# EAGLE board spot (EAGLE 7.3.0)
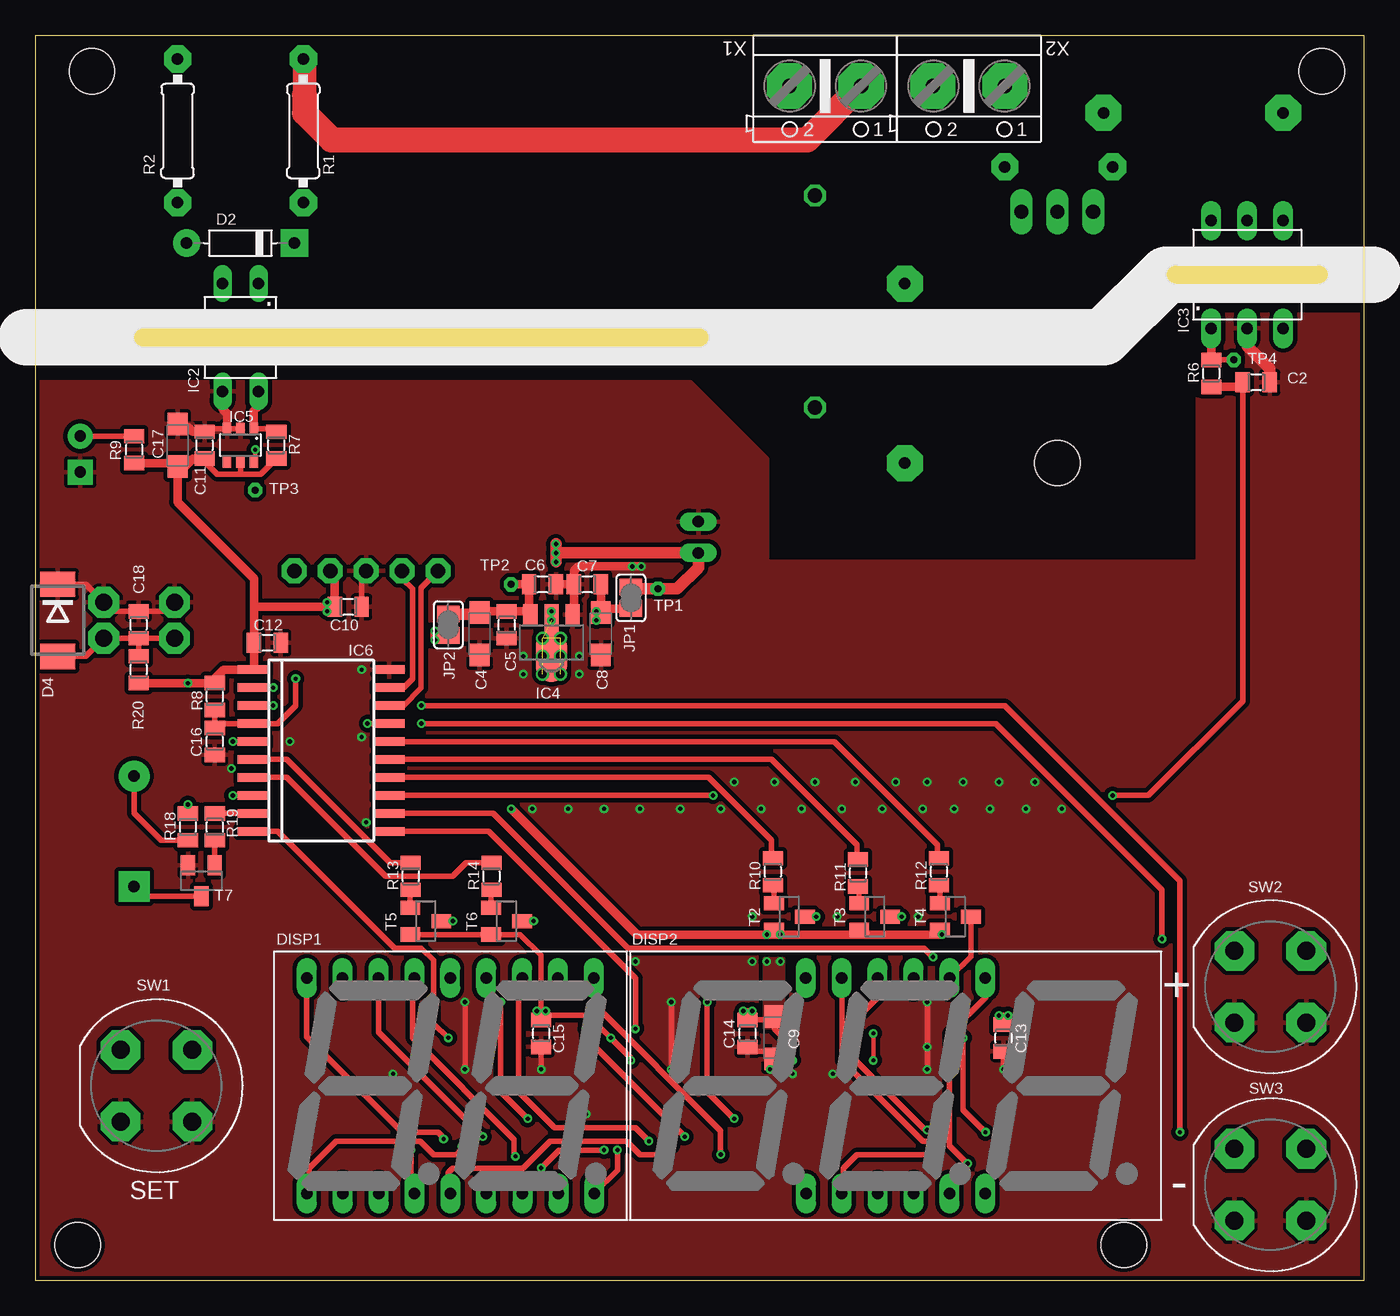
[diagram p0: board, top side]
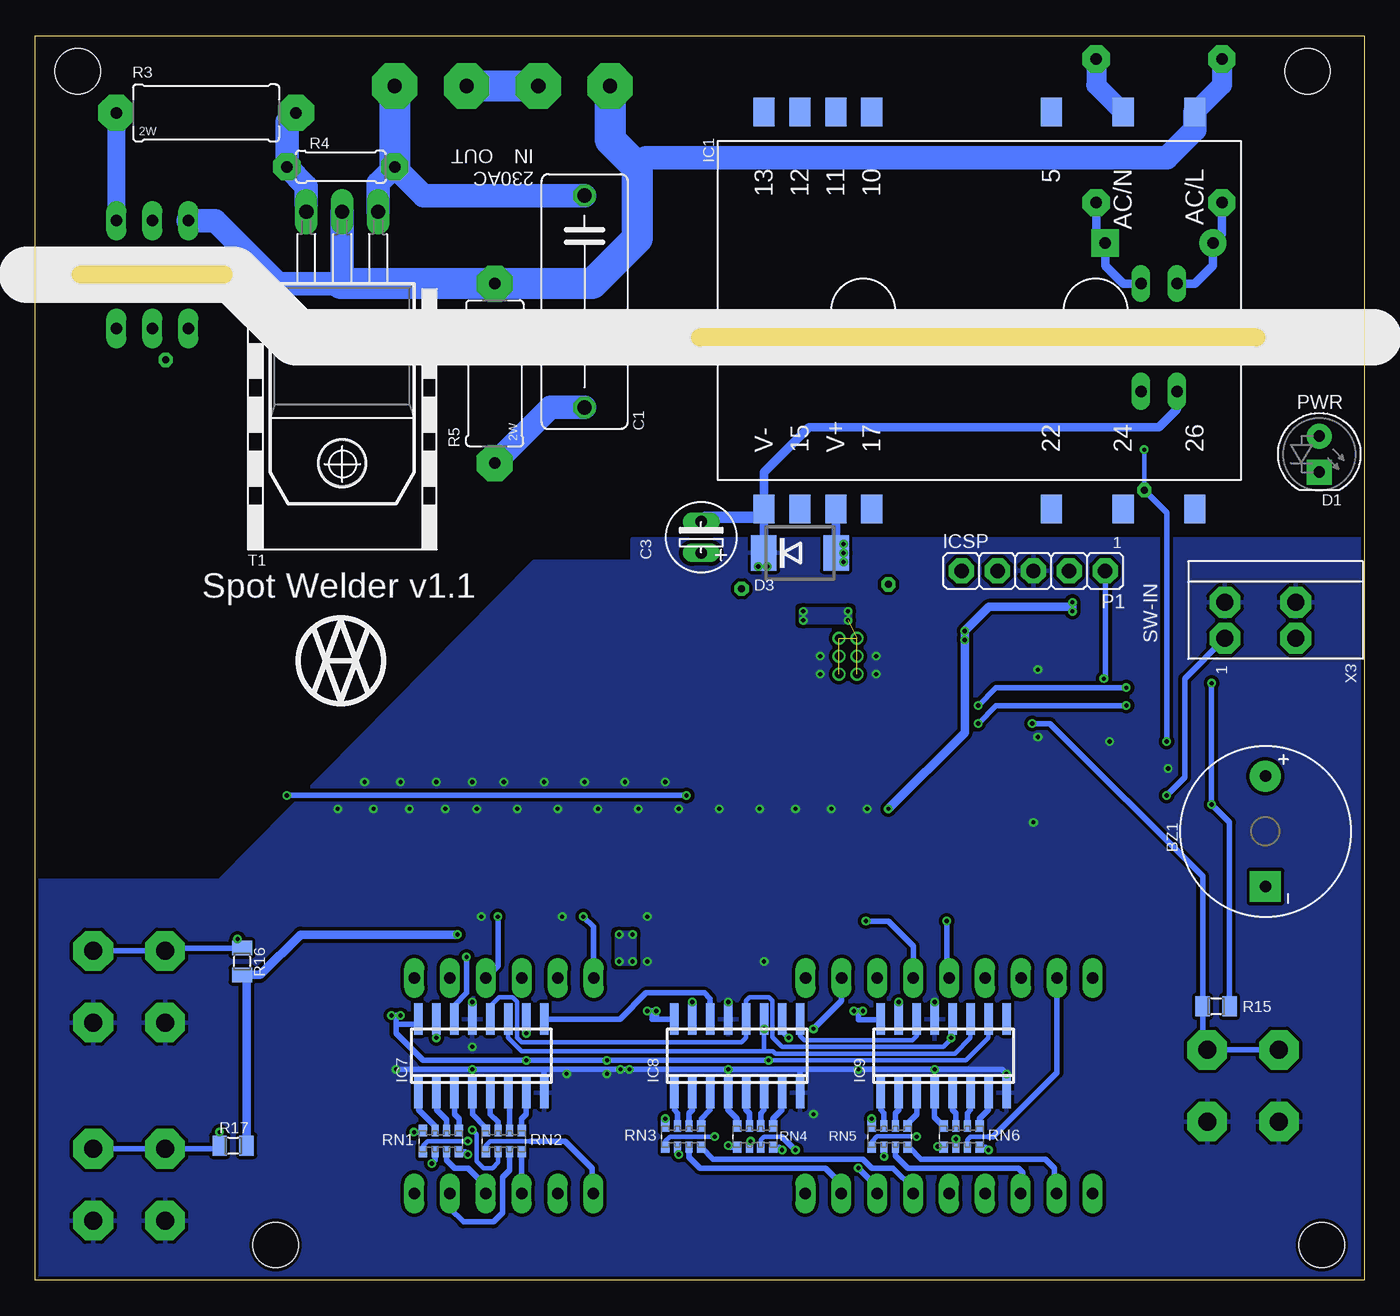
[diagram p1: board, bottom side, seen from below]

Size 94 x 88 mm. Coordinates in mm from the lower left corner, seen from the top.
Outline: 0,0 94,0 94,88 0,88 0,0
Copper layers (1*16): Top 0.035mm / dielectric 1.5mm / Bottom 0.035mm
Design rules "ITEADstudio_DRC": minimum track width 6mil, minimum drill 12mil, track to track 6mil, track to pad 6mil, pad to pad 6mil, via to via 6mil, smd to smd 0mil, copper to edge 10mil, drill to drill 10mil, minimum pad ring 10mil, minimum via ring 6mil, stop-mask expansion 2mil, vias tented up to drill 100mil, thermal gap 10mil
Holes 3.2 mm at 4,85.5 77,2.5 3,2.5 91,85.5 72.3,57.8
Milling: 2 lines

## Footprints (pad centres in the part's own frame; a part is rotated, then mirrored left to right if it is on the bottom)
BZEG1205 = drill 0.813 pad 2.184: + -3.9,0 | drill 0.813 pad 2.184 square: - 3.9,0
C150-064X183 = drill 1.016 octagon: 1 -7.493,0; 2 7.493,0
0805 = smd 1.016 x 1.422: 1 -0.953,0; 2 0.953,0
C-EL_2 = drill 0.813 pad 1.27 long: C+ 0,0; C- 2.223,0
SMC_A = smd 1.6 x 1.4: + -1.5,0; - 1.5,0
LED_5 = drill 0.813 pad 1.778: A -1.27,0 | drill 0.813 pad 1.778 square: K 1.27,0
DO35 = drill 0.813 pad 1.93: A -3.81,0 | drill 0.813 pad 1.93 square: K 3.81,0
DO214AA = smd 1.8 x 2.5: A 2.55,0; K -2.55,0
OPD-2 = drill 0.813 pad 1.4 long: 1 -10.16,-7.62; 2 -7.62,-7.62; 3 -5.08,-7.62; 4 -2.54,-7.62; 5 0,-7.62; 6 2.53,-7.62; 7 5.09,-7.62; 8 7.63,-7.62; 9 10.17,-7.62; 10 10.15,7.62; 11 7.61,7.62; 12 5.07,7.62; 13 2.53,7.62; 14 -0.01,7.62; 15 -2.55,7.62; 16 -5.09,7.62; 17 -7.63,7.62; 18 -10.17,7.62
OPD-3 = drill 0.813 pad 1.4 long: 1 -6.35,-7.62; 2 -3.81,-7.62; 3 -1.27,-7.62; 4 1.27,-7.62; 5 3.81,-7.62; 6 6.34,-7.62; 7 6.34,7.62; 8 3.8,7.62; 9 1.26,7.62; 10 -1.28,7.62; 11 -3.82,7.62; 12 -6.36,7.62
IRM_03_SMD = smd 1.5 x 2.03: 5 -5.08,-14.035; 10 7.62,-14.035; 11 10.16,-14.035; 12 12.7,-14.035; 13 15.24,-14.035; 15 12.7,14.035; 17 7.62,14.035; 22 -5.08,14.035; 24 -10.16,14.035; 26 -15.24,14.035; AC/L -15.24,-14.035; AC/N -10.16,-14.035; V+ 10.16,14.035; V- 15.24,14.035
DIL4 = drill 0.813 pad 1.27 long: 1 -1.27,-3.81; 2 1.27,-3.81; 3 1.27,3.81; 4 -1.27,3.81
DIL6 = drill 0.813 pad 1.4 long: 1 -2.54,-3.81; 2 0,-3.81; 3 2.54,-3.81; 4 2.54,3.81; 5 0,3.81; 6 -2.54,3.81
SOT89 = smd 1 x 1.5: 1 -1.499,-1.981; 3 1.499,-1.981 | smd 1 x 2: 2 0,-1.727 | smd 2.2 x 3.7: 2@1 0,0.94
SOT23-6 = smd 0.6 x 0.9: 1 -0.95,-1.15; 2 0,-1.15; 3 0.95,-1.15; 4 0.95,1.15; 5 0,1.15; 6 -0.95,1.15
SO-20 = smd 0.6 x 2.2: 1 -5.715,-4.8; 2 -4.445,-4.8; 3 -3.175,-4.8; 4 -1.905,-4.8; 5 -0.635,-4.8; 6 0.635,-4.8; 7 1.905,-4.8; 8 3.175,-4.8; 9 4.445,-4.8; 10 5.715,-4.8; 11 5.715,4.8; 12 4.445,4.8; 13 3.175,4.8; 14 1.905,4.8; 15 0.635,4.8; 16 -0.635,4.8; 17 -1.905,4.8; 18 -3.175,4.8; 19 -4.445,4.8; 20 -5.715,4.8
SO-16 = smd 0.6 x 2.2: 1 -4.445,-2.917; 2 -3.175,-2.917; 3 -1.905,-2.917; 4 -0.635,-2.917; 5 0.635,-2.917; 6 1.905,-2.917; 7 3.175,-2.917; 8 4.445,-2.917; 9 4.445,2.283; 10 3.175,2.283; 11 1.905,2.283; 12 0.635,2.283; 13 -0.635,2.283; 14 -1.905,2.283; 15 -3.175,2.283; 16 -4.445,2.283
JP = smd 1.168 x 1.6: 1 -0.762,0; 2 0.762,0
S5G1 = drill 1.016 pad 1.778 octagon: 1 -5.08,0; 2 -2.54,0; 3 0,0; 4 2.54,0; 5 5.08,0
R-10 = drill 0.813 pad 1.93 octagon: 1 -5.08,0; 2 5.08,0
R-_2W = drill 0.813 pad 2.54 octagon: 1 -6.35,0; 2 6.35,0
R-7,5 = drill 0.813 pad 1.93 octagon: 1 -3.81,0; 2 3.81,0
EXB38V = smd 0.6 x 0.8: 1 -1.275,-0.75; 4 1.275,-0.75; 5 1.275,0.75; 8 -1.275,0.75 | smd 0.5 x 0.8: 2 -0.4,-0.75; 3 0.4,-0.75; 6 0.4,0.75; 7 -0.4,0.75
P-DT6 = drill 1.27 pad 2.8 octagon: 1 -2.54,-2.54; 1A -2.54,2.54; 2 2.54,-2.54; 2A 2.54,2.54
TO-220 = drill 1.016 pad 1.6 long: 1 -2.54,0; 2 0,0; 3 2.54,0
SOT23 = smd 1 x 1.4: 1 -0.95,-1.1; 2 0.95,-1.1; 3 0,1.1
PAD_0,8 = drill 0.5 pad 0.813 octagon: 1 0,0
ARK500/2 = drill 1 pad 3.2 octagon: 1 -2.54,0; 2 2.54,0
DG240W = drill 1.2 pad 2.184 octagon: 1 -1.27,-2.54; 1_1 -1.27,2.46; 2 1.27,-2.54; 2_2 1.27,2.46

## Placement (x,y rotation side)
BZ1  BZEG-1205  [BZEG1205]  6.99,31.75 270 bottom
C1  100n/630  [C150-064X183]  55.15,69.22 270 bottom
C2  1n  [0805]  86.36,63.5 0 top
C3  47u/10  [C-EL_2]  46.9,51.44 90 bottom
C4  47u/6.3  [SMC_A]  31.43,45.72 270 top
C5  10u/10  [0805]  33.34,46.35 270 top
C6  100n  [0805]  35.88,49.21 0 top
C7  100n  [0805]  39.05,49.21 180 top
C8  10u/10  [SMC_A]  40.01,45.72 270 top
C9  10u/10  [SMC_A]  52.29,17.14 270 top
C10  100n  [0805]  22.13,47.62 0 top
C11  100n  [0805]  11.97,59.05 90 top
C12  100n  [0805]  16.41,45.09 0 top
C13  100n  [0805]  68.48,17.14 270 top
C14  100n  [0805]  50.39,17.46 270 top
C15  100n  [0805]  35.78,17.46 270 top
C16  100n  [0805]  12.7,38.1 270 top
C17  10u/10  [SMC_A]  10.06,59.05 90 top
C18  10n  [0805]  7.3,46.35 90 top
D1  [LED_5]  3.17,58.42 270 bottom
D2  1N4148  [DO35]  14.51,73.34 0 top
D3  P6SMBJ  [DO214AA]  39.91,51.44 0 bottom
D4  P6SMBJ  [DO214AA]  1.59,46.67 270 top
DISP1  OPD-D5630UPG  [OPD-2]  29.36,13.76 0 top
DISP2  OPD-T5620LE  [OPD-3]  60.87,13.76 0 top
IC1  [IRM_03_SMD]  27.21,68.58 180 bottom
IC2  PC817  [DIL4]  14.51,66.67 180 top
IC3  MOC3020  [DIL6]  85.72,71.12 0 top
IC4  MCP1702  [SOT89]  36.51,45.09 180 top
IC5  7417  [SOT23-6]  14.51,59.05 180 top
IC6  PIC16F18344SOIC  [SO-20]  20.23,37.47 270 top
IC7  74595SO  [SO-16]  62.45,16.19 0 bottom
IC8  74595SO  [SO-16]  44.35,16.19 0 bottom
IC9  74595SO  [SO-16]  29.75,16.19 0 bottom
JP1  JP  [JP]  42.13,48.26 90 top
JP2  JP  [JP]  29.21,46.35 270 top
KK1  D0A-L  [D02A-L]  72.3,63.18 90 bottom
P1  ICSP  [S5G1]  23.4,50.16 180 bottom
R1  100k  [R-10]  18.95,81.28 90 top
R2  100k  [R-10]  10.06,81.28 90 top
R3  1k  [R-_2W]  81.92,82.55 0 bottom
R4  330  [R-7,5]  72.39,78.74 180 bottom
R5  100  [R-_2W]  61.5,64.14 90 bottom
R6  1k  [0805]  83.19,64.14 90 top
R7  10k  [0805]  17.05,59.05 90 top
R8  10k  [0805]  12.7,41.27 90 top
R9  1k  [0805]  6.99,58.74 270 top
R10  2k  [0805]  52.17,28.89 90 top
R11  2k  [0805]  58.2,28.79 90 top
R12  2k  [0805]  63.92,28.89 90 top
R13  2k  [0805]  26.55,28.57 90 top
R14  2k  [0805]  32.27,28.57 90 top
R15  10k  [0805]  10.48,19.37 0 bottom
R16  10k  [0805]  79.38,22.54 270 bottom
R17  10k  [0805]  80.01,9.53 0 bottom
R18  220  [0805]  10.79,32.07 90 top
R19  10k  [0805]  12.7,32.07 270 top
R20  10k  [0805]  7.3,43.18 270 top
RN1  1k  [EXB38V]  65.31,9.84 0 bottom
RN2  1k  [EXB38V]  60.87,9.84 0 bottom
RN3  10k  [EXB38V]  48.16,10.16 0 bottom
RN4  10k  [EXB38V]  43.09,10.16 0 bottom
RN5  10k  [EXB38V]  33.56,10.16 0 bottom
RN6  10k  [EXB38V]  28.48,10.16 0 bottom
SW1  P-DT6  [P-DT6]  8.56,13.76 90 top
SW2  P-DT6  [P-DT6]  87.36,20.76 90 top
SW3  P-DT6  [P-DT6]  87.36,6.76 90 top
T1  BTA140  [TO-220]  72.3,75.56 180 bottom
T2  BC857  [SOT23]  53.34,25.72 270 top
T3  BC857  [SOT23]  59.37,25.72 270 top
T4  BC857  [SOT23]  65.09,25.72 270 top
T5  BC857  [SOT23]  27.62,25.4 270 top
T6  BC857  [SOT23]  33.34,25.4 270 top
T7  BC847  [SOT23]  11.75,28.26 180 top
TP1  PAD_10,8  [PAD_0,8]  44.04,48.9 0 top
TP2  PAD_10,8  [PAD_0,8]  33.66,49.21 0 top
TP3  PAD_10,8  [PAD_0,8]  15.56,55.88 0 top
TP4  PAD_10,8  [PAD_0,8]  84.77,65.09 0 top
U$1  [LOGO_AV3]  72.39,43.81 0 top
X1  AC IN  [ARK500/2]  55.88,84.45 180 top
X2  AC OUT  [ARK500/2]  66.04,84.45 180 top
X3  HANDLE  [DG240W]  7.3,46.67 270 bottom

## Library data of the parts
BZ1 C2 C3 C5-C7 C10-C16 C18 D1 IC2 R1-R20 T1 TP1-TP4 = #PaJa_31
C1 C4 C8 C9 C17 = rcl
D2 IC3 = #PaJa_30
D3 D4 IC4-IC9 JP1 JP2 P1 T2-T7 U$1 = !mcom2a
DISP1 DISP2 = #PaJa_displeje
IC1 = meanwell_irm_v7
KK1 = heatsink
RN1-RN6 = resistor-dil; OC_FARNELL: unknown; OC_NEWARK: unknown
SW1-SW3 = #PaJa_prepinace
X1-X3 = #PaJa_konektory

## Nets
!MCLR: C16.1 IC6.4 P1.1 R8.1
+3,3V: C9.+ C10.1 C11.1 C12.1 C13.1 C14.1 C15.1 C17.+ IC5.5 IC6.1 IC7.10 IC7.16 IC8.10 IC8.16 IC9.10 IC9.16 JP2.2 P1.2 R7.1 R8.2 R9.2 R15.2 R16.2 R17.2 R18.2 R20.2 T2.2 T3.2 T4.2 T5.2 T6.2
+5V: C3.C+ D3.A IC1.V+ JP1.2 TP1.1
BEEP: IC6.9 R19.1
CAD1_1: IC6.14 R10.2
CAD1_2: IC6.15 R11.2
CAD1_3: IC6.16 R12.2
CAD2_1: IC6.6 R13.2
CAD2_2: IC6.7 R14.2
D1_CA1: DISP2.12 T2.3
D1_CA2: DISP2.9 T3.3
D1_CA3: DISP2.8 T4.3
D2_CA1: DISP1.14 T5.3
D2_CA2: DISP1.13 T6.3
DS: IC6.12 IC7.14
GND: C2.2 C3.C- C4.- C5.2 C6.2 C7.2 C8.- C9.- C10.2 C11.2 C12.2 C13.2 C14.2 C15.2 C16.2 C17.- C18.2 D1.K D3.K D4.K IC1.V- IC2.3 IC3.2 IC4.1 IC5.2 IC5.3 IC6.20 IC7.8 IC7.13 IC8.8 IC8.13 IC9.8 IC9.13 P1.3 SW1.1 SW1.1A SW2.1 SW2.1A SW3.1 SW3.1A T7.2 X3.1 X3.1_1
INPUT: C18.1 D4.A IC6.8 R20.1 X3.2 X3.2_2
N$1: D2.K IC2.1 R1.1
N$2: D2.A IC2.2 R2.1
N$4: IC7.15 RN1.8
N$5: IC8.9 IC9.14
N$6: IC1.AC/L IC3.6 R2.2 R5.2 T1.2 X1.2
N$7: IC3.4 R3.1
N$8: R3.2 R4.2 T1.3
N$9: C1.1 R4.1 T1.1 X2.1
N$10: IC3.1 R6.2 TP4.1
N$11: C7.1 C8.+ IC4.2 JP1.1
N$12: C1.2 R5.1
N$13: C4.+ C5.1 C6.1 IC4.3 JP2.1 TP2.1
N$14: IC7.9 IC8.14
N$15: IC7.4 RN2.8
N$16: IC7.1 RN1.7
N$17: IC7.2 RN1.6
N$18: IC7.5 RN2.7
N$19: IC7.6 RN2.6
N$20: IC7.7 RN2.5
N$21: IC7.3 RN1.5
N$22: DISP2.11 RN1.1
N$23: DISP2.7 RN1.2
N$24: DISP2.4 RN1.3
N$25: DISP2.2 RN1.4
N$26: DISP2.1 RN2.1
N$27: DISP2.10 RN2.2
N$28: DISP2.5 RN2.3
N$29: DISP2.3 RN2.4
N$30: IC8.1 RN3.7
N$31: IC8.2 RN3.6
N$32: IC8.5 RN4.7
N$33: IC8.6 RN4.6
N$34: IC8.7 RN4.5
N$35: IC8.3 RN3.5
N$36: DISP1.16 RN5.1
N$37: DISP1.15 RN5.2
N$38: DISP1.3 RN5.3
N$39: DISP1.2 RN5.4
N$40: DISP1.1 RN6.1
N$41: DISP1.18 RN6.2
N$42: DISP1.17 RN6.3
N$43: DISP1.4 RN6.4
N$44: IC9.1 RN5.7
N$45: IC9.2 RN5.6
N$46: IC9.5 RN6.7
N$47: IC9.6 RN6.6
N$48: IC9.7 RN6.5
N$49: IC9.3 RN5.5
N$50: DISP1.11 RN3.1
N$51: DISP1.10 RN3.2
N$52: DISP1.8 RN3.3
N$53: DISP1.6 RN3.4
N$54: DISP1.5 RN4.1
N$55: DISP1.12 RN4.2
N$56: DISP1.7 RN4.3
N$57: DISP1.9 RN4.4
N$58: IC8.15 RN3.8
N$59: IC8.4 RN4.8
N$60: IC9.15 RN5.8
N$61: IC9.4 RN6.8
N$62: D1.A R9.1
N$63: R10.1 T2.1
N$64: R11.1 T3.1
N$65: R12.1 T4.1
N$66: R13.1 T5.1
N$67: R14.1 T6.1
N$68: BZ1.+ R18.1
N$69: BZ1.- T7.3
N$70: R19.2 T7.1
N$72: IC1.AC/N R1.2 X1.1 X2.2
N$74: IC2.4 IC5.1 R7.2
PGC: IC6.18 P1.5
PGD: IC6.19 P1.4
SCTP: IC6.10 IC7.12 IC8.12 IC9.12
SHCP: IC6.11 IC7.11 IC8.11 IC9.11
START: C2.1 IC6.13 R6.1
SW+: IC6.3 R16.1 SW2.2 SW2.2A
SW-: IC6.2 R17.1 SW3.2 SW3.2A
SW_P: IC6.17 R15.1 SW1.2 SW1.2A
ZERO: IC5.6 IC6.5 TP3.1

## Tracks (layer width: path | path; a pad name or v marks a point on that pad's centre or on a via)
!MCLR  (via drill 0.3)
  Top 0.406: R8.1 C16.1 13.02,39.37 IC6.4 17.14,39.37 18.41,40.64 v18.41,42.55
  Bottom 0.406: P1.1 18.32,42.64 v18.41,42.55
+3,3V  (via drill 0.3)
  Top 0.305: v59.28,17.46 v59.28,15.56
  Top 0.406: 36.1,18.73 v36.1,19.05 v35.47,19.05 35.76,19.05 35.77,19.06 35.77,22.97 34.29,24.45 T6.2 T5.2 | 36.1,18.73 35.78,18.73 C15.1 | v42.13,15.56 42.13,15.72 v40.7,17.14 39.12,18.73 36.1,18.73 | v50.7,19.05 v50.07,19.05 50.07,18.41 C14.1 52.06,18.41 C9.+ 52.29,17.78 53.56,16.51 v53.56,15.56 | v68.8,18.73 v68.17,18.73 68.48,18.73 C13.1 | JP2.2 28.57,45.59 v28.26,45.28 | R18.2 v10.79,33.66 | 17.05,58.01 R7.1 15.94,56.99 14.61,56.99 | IC5.5 14.51,57.09 14.61,56.99 | C11.1 11.97,57.88 12.86,56.99 14.61,56.99
  Top 0.61: v52.7,24.45 52.56,24.77 T2.2 | 52.07,18.87 C9.+ | C10.1 21.18,49.85 P1.2 | v28.26,45.92 v28.26,45.28 | C10.1 20.95,47.62 v20.64,47.94 v20.64,47.31 | 15.46,47.62 C10.1 | 15.46,47.62 C12.1 15.46,43.22 IC6.1 13.34,43.18 12.7,42.55 R8.2 v10.79,42.23 R20.2 | v33.66,33.34 42.55,24.45 v52.7,24.45 | T2.2 52.07,24.77 v51.75,24.45 | 15.46,47.62 15.46,49.62 10.06,55.02 C17.+ | T2.2 52.38,24.77 v52.7,24.45 | T4.2 63.99,24.45 v64.14,24.45 58.27,24.45 T3.2 58.27,24.59 58.42,24.45 v52.7,24.45 | C11.1 11.11,58.1 10.48,57.47 10.15,57.47 C17.+ | R9.2 9.84,57.78 C17.+
  Bottom 0.305: IC9.10 26.57,17.14 28.16,15.56 v42.13,15.56 | 41.18,19.21 IC8.10 41.08,18.57 41.08,17.68 | IC7.10 v59.28,17.46
  Bottom 0.406: v36.1,19.05 v35.47,19.05 35.78,19.05 C15.1 34.26,18.41 IC9.16 34.2,18.41 | 41.08,17.68 41.08,17.52 v40.7,17.14 | 50.39,19.05 v50.07,19.05 50.07,18.73 | 50.39,19.05 v50.7,19.05 | IC8.16 50.39,18.48 50.39,19.05 | C13.1 66.9,18.1 IC7.16 | C13.1 68.48,17.46 66.58,15.56 v59.28,15.56 v53.56,15.56 v42.13,15.56 | v68.17,18.73 68.48,18.73 | 68.48,18.73 v68.8,18.73 | C13.1 68.48,18.73 | v10.79,42.23 v10.79,33.66 | 10.48,33.34 v10.79,33.66 | R15.2 9.53,32.38 v10.79,33.66
  Bottom 0.61: v20.64,47.94 20.64,47.62 | 20.64,47.62 v20.64,47.31 | v28.26,45.92 28.26,45.4 | 20.64,47.62 26.55,47.62 v28.26,45.92 | v28.26,45.92 28.26,38.73 v33.66,33.34 | R17.2 79.06,21.27 R16.2 78.11,21.59 75.25,24.45 v64.14,24.45
  other vias: 51.75,22.54 52.7,22.54
  pour Bottom: 51.75,24.45 51.75,22.54 52.7,22.54 52.7,24.45
  pour Top (no thermals): 51.5,22.8 53,22.8 53,17.8 51.5,17.8
+5V  (via drill 0.3)
  Top 0.813: v36.83,51.44 v36.83,50.8 | v36.83,52.07 v36.83,51.44 | JP1.2 42.26,48.9 TP1.1 45.4,48.9 46.9,50.39 C3.C+ v36.83,51.44
  Bottom 0.61: IC1.V+ D3.A
  Bottom 0.813: 37.47,52.07 37.47,51.44 D3.A v36.83,51.44
BEEP
  Top 0.406: R19.1 IC6.9
CAD1_1
  Top 0.406: R10.2 52.07,29.95 52.07,31.11 47.62,35.56 IC6.14
CAD1_2
  Top 0.406: R11.2 58.1,29.84 58.1,30.8 52.07,36.83 IC6.15
CAD1_3
  Top 0.406: R12.2 63.82,29.95 63.82,30.8 56.52,38.1 IC6.16
CAD2_1
  Top 0.406: R13.2 25.08,29.53 17.78,36.83 IC6.6
CAD2_2
  Top 0.406: R14.2 30.48,29.53 29.53,28.57 24.77,28.57 17.78,35.56 IC6.7
D1_CA1  (via drill 0.3)
  Top 0.406: v55.24,25.72 T2.3
  Bottom 0.406: DISP2.12 54.52,25 v55.24,25.72
D1_CA2  (via drill 0.3)
  Top 0.406: v61.28,25.72 T3.3
  Bottom 0.406: v61.28,25.72 61.28,22.25 DISP2.9
D1_CA3
  Top 0.406: T4.3 66.19,22.89 DISP2.8
D2_CA1  (via drill 0.3)
  Top 0.406: v29.53,25.4 T5.3
  Bottom 0.406: v29.53,25.4 29.53,21.55 DISP1.14
D2_CA2  (via drill 0.3)
  Top 0.406: v35.24,25.4 T6.3
  Bottom 0.406: DISP1.13 31.89,23.64 33.66,25.4 v35.24,25.4
DS  (via drill 0.3)
  Top 0.406: v63.5,22.86 62.87,23.5 41.91,23.5 32.38,33.02 IC6.12
  Bottom 0.406: v63.5,22.86 63.5,20.32 64.36,19.46 IC7.14
GND  (via drill 0.3)
  Top 0.406: v44.99,19.68 v44.99,14.92 | v30.39,19.68 v30.39,14.92 | C15.2 v35.78,14.92 | v63.09,19.68 v63.09,14.92 | C13.2 v68.48,14.92 | C14.2 50.7,16.51 51.02,16.19 51.74,16.19 C9.- 52.61,15.33 v52.61,14.92 v51.98,14.92 | C10.2 23.08,49.85 P1.3 | X3.1 9.21,47.31 C18.2 5.48,47.31 X3.1_1 3.56,49.22 D4.K | IC5.2 IC5.3 12.17,60.2 C11.2
  Top 0.61: C7.2 C6.2 | C7.2 38.1,47.15 IC4.1 | v42.86,50.48 38.42,50.48 38.1,50.16 C7.2 | IC5.3 13.56,61.27 13.24,61.59 IC2.3 | C11.2 11.11,60.01 10.79,60.33 10.29,60.33 C17.-
  Top 0.813: IC3.2 85.72,66.04 87.31,64.45 C2.2
  Bottom 0.406: IC8.13 v44.99,19.68 | IC9.13 v30.39,19.68 | IC7.13 v63.09,19.68 | v68.48,14.92 v63.09,14.92 58.01,14.92 | 58.01,14.92 v51.98,14.92 v44.99,14.92 39.91,14.92 | 39.91,14.92 v35.78,14.92 v30.39,14.92 25.62,14.92 v25.3,14.61 IC9.8 | IC8.8 39.91,14.92 | IC7.8 58.01,14.92
  Bottom 0.61: IC2.3 13.24,61.59 14.51,60.33 39.27,60.33 42.45,57.15 IC1.V- 42.45,53.98 D3.K | D3.K | D3.K 42.45,50.9 v42.86,50.48
  Bottom 0.813: 42.45,53.98 46.58,53.98 C3.C-
  other vias: 42.23,50.48 56.42,14.61 53.56,14.61 38.96,11.75 63.09,16.51 23.4,32.38 23.08,38.42 18,38.1 23.08,43.18 34.51,44.13 34.51,42.86 38.48,42.86 38.48,44.13 50.7,25.72 56.74,25.72 62.45,25.72 13.88,36.2 72.61,33.34 70.71,35.24 70.07,33.34 68.17,35.24 67.53,33.34 65.63,35.24 64.99,33.34 63.09,35.24 62.77,33.34 60.87,35.24 59.91,33.34 58.01,35.24 57.05,33.34 55.15,35.24 54.2,33.34 52.29,35.24 51.34,33.34 49.44,35.24 48.48,33.34 45.62,33.34 42.77,33.34 40.23,33.34 37.69,33.34 35.15,33.34 50.7,22.54 42.45,22.54
  pour Top (isolate 0.305, rank 2): 93.98,68.26 82.23,68.26 82.23,50.8 51.75,50.8 51.75,58.1 46.35,63.5 0,63.5 0,0 93.98,0
  pour Bottom (isolate 0.254, rank 2): 0,52.39 51.75,52.39 51.75,50.8 58.74,50.8 80.96,28.26 93.98,28.26 93.98,0 0,0
INPUT  (via drill 0.3)
  Top 0.406: C18.1 R20.1 | C18.1 X3.2_2 3.56,44.12 D4.A | IC6.8 v13.97,34.29 | C18.1 X3.2
  Bottom 0.406: v13.97,34.29 12.7,35.56 12.7,42.55 X3.2
N$1
  Bottom 0.61: IC2.1 17.05,70.48 18.32,71.75 D2.K 18.95,73.98 R1.1
N$2
  Bottom 0.61: IC2.2 11.97,70.48 10.7,71.75 D2.A 10.06,73.98 R2.1
N$4  (via drill 0.3)
  Top 0.406: v65.63,17.14 65.63,12.06 v67.22,10.48
  Bottom 0.406: IC7.15 v65.63,17.14 | v67.22,10.48 66.7,10.48 RN1.8
N$5
  Bottom 0.305: IC8.9 39.91,17.3 39.59,16.99 31.97,16.99 31.66,17.3 IC9.14
N$6
  Bottom 1.422: R2.2 10.06,84.52 IC1.AC/L
  Bottom 1.676: IC1.AC/L 11.97,81.38 13.97,79.38 50.8,79.38 51.44,78.74 | 72.3,70.48 72.39,70.48 | 72.39,70.48 76.83,70.48 81.28,74.93 IC3.6 | T1.2 72.3,70.58 72.39,70.48
  Bottom 2.184: 72.39,70.48 R5.2 54.61,70.48 51.44,73.66 51.44,78.74 53.34,80.64 X1.2
N$7
  Bottom 1.27: R3.1 IC3.4
N$8
  Bottom 1.27: T1.3 74.83,76.11
  Bottom 1.676: 74.83,76.11 74.83,77.38 R4.2 76.2,81.92 R3.2
N$9
  Bottom 1.676: C1.1 66.55,76.71 R4.1 69.75,77.56 T1.1
  Bottom 2.184: X2.1 R4.1
N$10
  Top 0.406: TP4.1 R6.2
  Top 0.61: IC3.1 R6.2
N$11  (via drill 0.3, 0.6)  (6 unrouted)
  Top 0.61: C7.1 40.01,47.54 v39.69,47.31 C8.+ 40.28,47.5 JP1.1 | IC4.2 v36.51,46.67
  other vias: 36.51,47.31 39.69,46.67 35.88,45.4 37.15,45.4 35.88,44.13 37.15,44.13 35.88,42.86 37.15,42.86
  pour Bottom: 36.51,47.31 39.69,47.31 39.69,46.67 36.51,46.67
N$12
  Bottom 1.676: C1.2 57.56,61.72 R5.1
N$13
  Top 0.61: C4.+ 31.74,47.31 C5.1 34.99,47.31 IC4.3 34.92,47.15 C6.1 TP2.1
  Top 0.813: JP2.1 31.33,47.12 C4.+
N$14
  Bottom 0.406: IC7.9 52.65,18.48 50.8,20.32 46.67,20.32 46.26,19.91 IC8.14
N$15
  Bottom 0.406: RN2.8 62.14,10.8 63.09,11.75 IC7.4
N$16
  Bottom 0.406: RN1.7 65.71,10.88 66.9,12.06 IC7.1
N$17
  Bottom 0.406: IC7.2 65.63,12.06 64.91,11.35 RN1.6
N$18
  Bottom 0.406: RN2.7 61.27,11.2 61.82,11.75 IC7.5
N$19
  Bottom 0.406: RN2.6 60.47,13.19 IC7.6
N$20
  Bottom 0.406: RN2.5 59.59,11.44 59.28,11.75 IC7.7
N$21
  Bottom 0.406: IC7.3 64.36,11.75 64.04,11.43 RN1.5
N$22  (via drill 0.3)
  Top 0.406: v63.41,9.84 62.77,9.84 57.06,15.55 DISP2.11
  Bottom 0.305: RN1.1 66.58,9.52 66.26,9.84 v63.41,9.84
N$23  (via drill 0.3)
  Top 0.406: v65.94,8.26 64.67,9.53 64.67,17.46 67.22,20.01 DISP2.7
  Bottom 0.406: RN1.2 65.71,8.49 v65.94,8.26
N$24
  Bottom 0.406: RN1.3 64.91,8.49 64.36,7.94 63.41,7.94 62.16,6.69 DISP2.4
N$25  (via drill 0.3)
  Top 0.406: v63.41,8.89 58.1,8.89 57.15,7.94 57.15,6.22 DISP2.2
  Bottom 0.406: RN1.4 63.61,9.09 v63.41,8.89
N$26
  Bottom 0.305: RN2.1 62.14,9.52 61.82,9.84 58.96,9.84
  Bottom 0.406: 58.96,9.84 56.52,9.84 54.61,7.94 54.61,6.22 DISP2.1
N$27  (via drill 0.3)
  Top 0.406: v63.09,10.64 62.93,10.64 58.01,15.56 58.01,18.41 59.6,20.01 DISP2.10
  Bottom 0.305: RN2.2 61.27,8.33 61.66,7.94 62.29,7.94 62.77,8.41 62.77,10.32 v63.09,10.64
N$28
  Bottom 0.406: DISP2.5 64.69,5.1 63.72,4.13 61.59,4.13 60.96,4.76 60.96,7.3 60.47,7.8 RN2.3
N$29
  Bottom 0.406: RN2.4 59.59,6.38 DISP2.3
N$30
  Bottom 0.406: RN3.7 48.56,11.83 48.8,12.06 IC8.1
N$31
  Bottom 0.406: RN3.6 47.77,11.83 47.53,12.06 IC8.2
N$32
  Bottom 0.406: RN4.7 43.48,11.83 43.72,12.06 IC8.5
N$33
  Bottom 0.406: RN4.6 42.69,11.83 42.45,12.06 IC8.6
N$34
  Bottom 0.406: IC8.7 41.18,12.06 41.81,11.43 RN4.5
N$35
  Bottom 0.406: RN3.5 46.89,11.44 46.26,12.06 IC8.3
N$36  (via drill 0.3)
  Top 0.406: DISP1.16 24.27,17.54 v31.66,10.16
  Bottom 0.305: RN5.1 34.84,9.8 34.47,10.17 v31.66,10.17 v31.66,10.16
N$37  (via drill 0.3)
  Top 0.406: 33.96,8.88 v33.97,8.77 33.88,8.86 33.88,9.94 26.67,17.14 26.67,21.25 DISP1.15
  Bottom 0.406: v33.97,8.77 RN5.2
N$38
  Bottom 0.406: RN5.3 33.16,8.81 32.29,7.94 24.45,7.94 24.13,7.62 24.13,6.3 DISP1.3
N$39
  Bottom 0.406: RN5.4 32.17,9.41 31.34,8.57 22.54,8.57 21.91,7.94 21.91,6.31 DISP1.2
N$40  (via drill 0.3)
  Top 0.406: v30.16,9.47 30.16,9.3 29.75,8.89 28.16,8.89 27.21,9.84 21.27,9.84 19.37,7.94 19.37,6.31 DISP1.1
  Bottom 0.406: RN6.1 30.11,9.41 v30.16,9.47
N$41  (via drill 0.3)
  Top 0.406: v28.88,9.98 28.88,10.08 28.48,10.48 25.94,10.48 19.2,17.22 DISP1.18
  Bottom 0.406: RN6.2 v28.88,9.98 28.86,9.87
N$42
  Bottom 0.305: RN6.3 28.08,9.93 27.84,10.16 26.57,10.16
  Bottom 0.406: 26.57,10.16 26.26,10.16 21.73,14.68 DISP1.17
N$43  (via drill 0.3)
  Top 0.406: v26.57,9.21 26.57,6.4 DISP1.4
  Bottom 0.406: RN6.4 26.78,9.41 v26.57,9.21
N$44
  Bottom 0.406: RN5.7 33.96,11.83 34.2,12.06 IC9.1
N$45
  Bottom 0.406: RN5.6 33.16,11.83 32.92,12.06 IC9.2
N$46
  Bottom 0.406: RN6.7 28.88,11.83 29.11,12.06 IC9.5
N$47
  Bottom 0.406: RN6.6 28.08,11.83 27.84,12.06 IC9.6
N$48
  Bottom 0.406: RN6.5 27.2,11.44 26.57,12.06 IC9.7
N$49
  Bottom 0.406: RN5.5 32.28,11.12 31.66,11.75 IC9.3
N$50  (via drill 0.3)
  Top 0.406: v45.94,10.16 38.96,17.14 v38.96,17.78
  Bottom 0.305: RN3.1 49.44,9.84 49.12,10.16 v45.94,10.16
  Bottom 0.406: DISP1.11 36.98,19.76 v38.96,17.78
N$51  (via drill 0.3)
  Top 0.406: v48.48,8.89 48.48,10.57 39.52,19.54 DISP1.10
  Bottom 0.406: RN3.2 48.56,8.97 v48.48,8.89
N$52
  Bottom 0.406: DISP1.8 36.99,6.83 38.1,7.94 46.99,7.94 47.77,8.71 RN3.3
N$53
  Bottom 0.406: 46.78,9.41 RN3.4 46.05,8.57 35.47,8.57 34.83,7.94 33.34,7.94 31.89,6.5 DISP1.6
N$54  (via drill 0.3)
  Top 0.406: v44.99,9.53 44.35,8.89 42.77,8.89 41.81,9.84 36.42,9.84 34.51,7.94 29.53,7.94 29.21,7.62 29.21,6.3 DISP1.5
  Bottom 0.406: RN4.1 44.79,9.41 v44.99,9.53
N$55  (via drill 0.3)
  Top 0.406: v43.4,9.84 42.45,10.79 36.73,10.79 34.2,13.34 34.2,21.15 DISP1.12
  Bottom 0.406: RN4.2 43.48,9.76 v43.4,9.84
N$56  (via drill 0.3)
  Top 0.406: v40.23,9.21 37.05,9.21 v35.78,7.94
  Bottom 0.305: RN4.3 42.69,9.93 42.45,10.16 41.18,10.16
  Bottom 0.406: v40.23,9.21 41.18,10.16 | DISP1.7 34.45,6.61 v35.78,7.94
N$57  (via drill 0.3)
  Top 0.406: v41.18,9.21 41.18,7.79 DISP1.9
  Bottom 0.406: RN4.4 41.38,9.41 v41.18,9.21
N$58  (via drill 0.3)
  Top 0.406: v47.53,19.68 47.53,13.34 v49.44,11.43
  Bottom 0.406: IC8.15 v47.53,19.68 | v49.44,11.43 RN3.8
N$59
  Bottom 0.406: IC8.4 44.99,12.06 44.35,11.43 RN4.8
N$60  (via drill 0.3)
  Top 0.406: v32.92,19.68 32.92,13.34 v34.83,11.43
  Bottom 0.406: IC9.15 v32.92,19.68 | RN5.8 v34.84,11.43 v34.83,11.43 RN5.8
N$61
  Bottom 0.406: IC9.4 30.39,11.54 RN6.8
N$62
  Top 0.406: R9.1 D1.A
N$63
  Top 0.406: 52.07,26.84 T2.1 52.24,27.94 R10.1
N$64
  Top 0.406: 58.1,26.84 T3.1 58.27,27.84 R11.1
N$65
  Top 0.406: 63.82,26.84 T4.1 63.99,27.94 R12.1
N$66
  Top 0.406: 26.35,26.5 T5.1 26.52,27.62 R13.1
N$67
  Top 0.406: 32.07,26.52 T6.1 32.24,27.62 R14.1
N$68
  Top 0.406: R18.1 8.89,31.11 6.99,33.02 BZ1.+
N$69
  Top 0.406: T7.3 7.68,27.16 BZ1.-
N$70
  Top 0.406: T7.1 R19.2
N$72
  Top 1.676: 19.05,83.82 19.05,86.27 R1.2
  Top 1.778: 19.05,83.82 19.05,82.55 20.95,80.64 54.61,80.64 X1.1
  Bottom 1.422: R1.2 18.95,84.52 IC1.AC/N
  Bottom 2.184: X2.2 X1.1
N$74
  Top 0.406: IC5.1 16.85,60.2 R7.2
  Top 0.61: IC2.4 15.78,61.82 15.46,61.5 IC5.1
PGC
  Top 0.406: IC6.18 26.04,40.64 27.3,41.91 27.3,48.99 P1.5
PGD
  Top 0.406: IC6.19 26.04,41.91 26.67,42.55 26.67,48.9 25.94,49.62 P1.4
SCTP  (via drill 0.3)
  Top 0.406: v29.21,17.14 29.18,17.14 28.16,18.16 28.16,22.64 27.3,23.5 25.4,23.5 17.14,31.75 IC6.10
  Bottom 0.305: IC9.12 29.11,17.14 29.75,16.51 41.18,16.51 41.87,17.2 41.87,19.76 42.11,20 43.5,20 43.72,19.78 IC8.12 43.72,17.14 44.04,16.83 59.59,16.83 59.91,17.14 59.91,19.68 60.23,20 61.18,20 61.82,19.37 IC7.12
  Bottom 0.406: IC9.12 29.11,17.24 v29.21,17.14
SHCP  (via drill 0.3)
  Top 0.406: 42.55,17.88 v42.45,17.78 42.45,21.37 32.07,31.75 IC6.11
  Bottom 0.305: IC9.11 27.84,17.14 28.96,16.03 41.66,16.03 41.81,16.19 42.45,16.19 | 42.45,16.19 59.59,16.19 60.55,17.14 IC7.11 | 42.45,16.19 v42.45,17.78 IC8.11
START  (via drill 0.3)
  Top 0.406: v76.2,34.29 78.74,34.29 85.41,40.96 C2.1 | IC6.13 v47.94,34.29
  Top 0.61: R6.1 85,63.18 C2.1
  Bottom 0.406: v47.94,34.29 v76.2,34.29
SW+  (via drill 0.3)
  Top 0.406: IC6.3 v16.83,40.64 | v79.69,24.13 79.69,27.62 67.94,39.37 v27.3,39.37
  Bottom 0.406: SW2.2 SW2.2A 84.63,23.5 R16.1 v79.69,24.13 | v16.83,40.64 26.04,40.64 v27.3,39.37
SW-  (via drill 0.3)
  Top 0.406: IC6.2 v16.83,41.91 | v80.96,10.48 80.96,28.26 68.58,40.64 v27.3,40.64
  Bottom 0.406: v80.96,10.48 R17.1 81.19,9.3 SW3.2A SW3.2 | v16.83,41.91 26.04,41.91 v27.3,40.64
SW_P  (via drill 0.3)
  Top 0.406: IC6.17 v23.5,39.37
  Bottom 0.406: SW1.2A SW1.2 11.43,16.61 R15.1 11.43,28.57 22.23,39.37 v23.5,39.37
ZERO  (via drill 0.3)
  Top 0.305: 15.48,58.02 IC5.6 15.56,58.16 v15.56,58.74
  Top 0.406: v13.97,38.1 IC6.5
  Bottom 0.305: v15.56,58.74 TP3.1
  Bottom 0.406: v13.97,38.1 13.97,54.29 TP3.1

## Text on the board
tNames: . | . | + | SET | -
bNames: IN | OUT | 230AC | PWR | 1 | ICSP | Spot Welder v1.1 | SW-IN | 1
